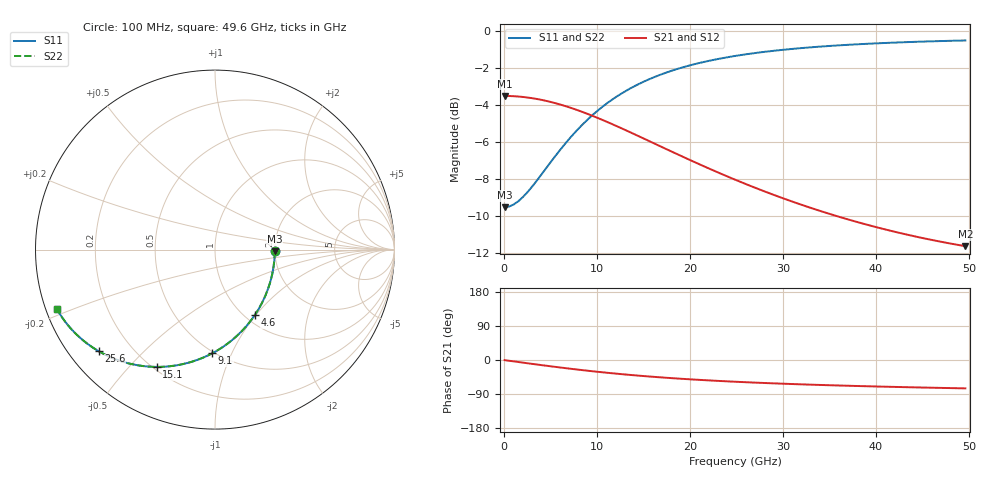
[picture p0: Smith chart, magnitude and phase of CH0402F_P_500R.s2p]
# GHz S RI R 500
! S-Parameters data
! Freq  reS11  imS11  reS21  imS21  reS12  imS12  reS22  imS22
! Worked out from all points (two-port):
!   100 points, 100 MHz to 49.6 GHz, reference 500 ohm
!   highest |S21| = -3.52 dB at 100 MHz (marker M1); lowest = -11.6 dB at 49.6 GHz (marker M2)
!   |S21| within 3 dB of the highest: start of sweep to 18.03 GHz
!   lowest |S11| = -9.5 dB at 100 MHz (marker M3), VSWR 2.00, Z = 1e+03 - j19.5 ohm
!   |S11| at or under -10 dB: nowhere
!   |S22| runs from -9.5 to -0.5 dB; largest |S21 - S12| = 0
!   S11 on the Smith chart (normalised r, x): 100 MHz: 2.00, -0.04; 4.6 GHz: 1.11, -0.99; 9.1 GHz: 0.49, -0.85; 15.1 GHz: 0.21, -0.60; 25.6 GHz: 0.09, -0.37; 49.6 GHz: 0.03, -0.18
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0.1  0.3333 -0.00865  0.6666 -0.00392  0.6666 -0.00392  0.3333 -0.00865
1.1  0.3264 -0.0947  0.6641 -0.0429  0.6641 -0.0429  0.3264 -0.0947
2.1  0.3085 -0.1782  0.6573 -0.0811  0.6573 -0.0811  0.3085 -0.1782
3.1  0.2804 -0.2574  0.6465 -0.118  0.6465 -0.118  0.2804 -0.2574
4.6  0.2222 -0.3642  0.6236 -0.1693  0.6236 -0.1693  0.2222 -0.3642
6.6  0.1234 -0.4796  0.5831 -0.2281  0.5831 -0.2281  0.1234 -0.4796
8.6  0.0125 -0.5622  0.5355 -0.2743  0.5355 -0.2743  0.0125 -0.5622
9.1  -0.0157 -0.578  0.523 -0.2838  0.523 -0.2838  -0.0157 -0.578
10.6  -0.0995 -0.6149  0.485 -0.3078  0.485 -0.3078  -0.0995 -0.6149
12.1  -0.1798 -0.6382  0.4473 -0.3254  0.4473 -0.3254  -0.1798 -0.6382
15.1  -0.3241 -0.6536  0.3767 -0.345  0.3767 -0.345  -0.3241 -0.6536
16.6  -0.3869 -0.6503  0.3448 -0.3488  0.3448 -0.3488  -0.3869 -0.6503
18.6  -0.461 -0.6385  0.3064 -0.3495  0.3064 -0.3495  -0.461 -0.6385
20.6  -0.5249 -0.6211  0.2725 -0.3465  0.2725 -0.3465  -0.5249 -0.6211
22.6  -0.5798 -0.6003  0.2428 -0.3412  0.2428 -0.3412  -0.5798 -0.6003
25.1  -0.6375 -0.5719  0.2111 -0.3326  0.2111 -0.3326  -0.6375 -0.5719
25.6  -0.6478 -0.5661  0.2053 -0.3307  0.2053 -0.3307  -0.6478 -0.5661
29.1  -0.7099 -0.5251  0.1704 -0.3169  0.1704 -0.3169  -0.7099 -0.5251
33.1  -0.7639 -0.48  0.1395 -0.3011  0.1395 -0.3011  -0.7639 -0.48
37.1  -0.8047 -0.4381  0.1156 -0.2865  0.1156 -0.2865  -0.8047 -0.4381
41.6  -0.8394 -0.3952  0.0948 -0.2722  0.0948 -0.2722  -0.8394 -0.3952
49.6  -0.8817 -0.3289  0.0684 -0.253  0.0684 -0.253  -0.8817 -0.3289
